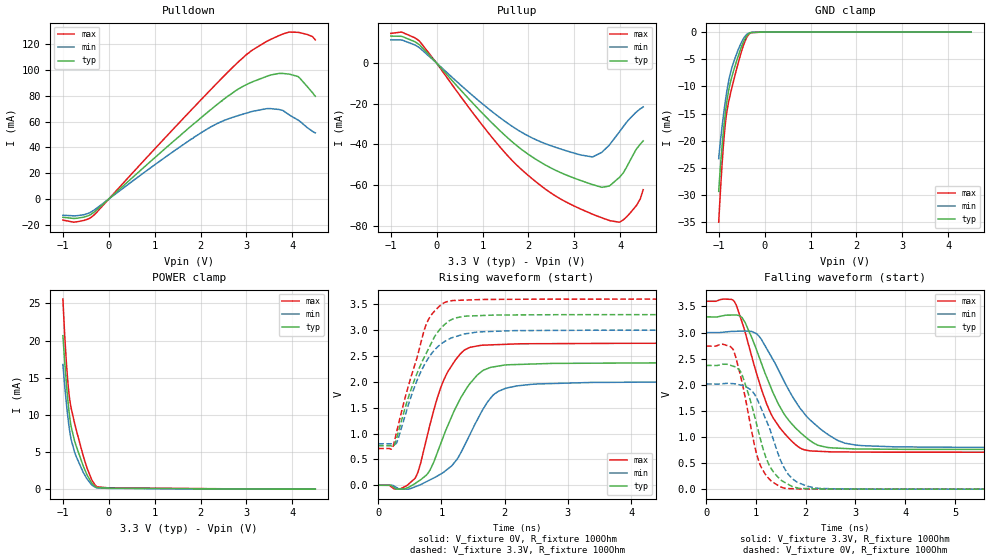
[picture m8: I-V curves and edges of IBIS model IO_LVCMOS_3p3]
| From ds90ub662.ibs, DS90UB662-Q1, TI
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|   IO_LVCMOS_3p3 Model
[Model]   IO_LVCMOS_3p3
Model_type   I/O
Polarity   Non-Inverting
Enable   Active-Low
Vinl = 0.99
Vinh = 2.31
Vmeas = 1.65
Vref = 0
Cref = 1pF
Rref = 100000
|   typ   min   max
C_comp   0.362pF   0.313pF   0.461pF
[Voltage Range]   3.3   3   3.6
[Temperature Range]   27   105   -40
[Pullup Reference]   3.3   3   3.6
[Pulldown Reference]   0   0   0
[Power Clamp Reference]   3.3   3   3.6
[GND Clamp Reference]   0   0   0
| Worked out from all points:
|   slope of the pulldown table from 0 to 0.495 V, typ, clamps not added: 31.1 ohm
|   slope of the pullup table from 0 to 0.495 V, typ, clamps not added: 39.6 ohm
|   GND clamp passes 1 mA (typ) near -0.41 V on its own axis
|   POWER clamp passes 1 mA (typ) near -0.39 V on its own axis
|   falling waveform, V_fixture 3.3V, R_fixture 100Ohm: 20-80 % time 741ps typ, 895ps min, 623ps max; typ from 3.3 V to 0.76 V
|   rising waveform, V_fixture 0V, R_fixture 100Ohm: 20-80 % time 524ps typ, 549ps min, 407ps max; typ from 0 V to 2.37 V
|   rising waveform, V_fixture 3.3V, R_fixture 100Ohm: 20-80 % time 485ps typ, 453ps min, 391ps max; typ from 0.764 V to 3.3 V
|   falling waveform, V_fixture 0V, R_fixture 100Ohm: 20-80 % time 435ps typ, 495ps min, 369ps max; typ from 2.37 V to 0 V
[Pulldown]
|   Voltage   I(typ)   I(min)   I(max)
-1V       -14.12mA   -12.57mA   -16.32mA
-686.5mV  -14.88mA   -12.9mA    -17.62mA
-318mV    -10.15mA   -8.516mA   -12.27mA
1.855V    58.36mA    47.77mA    71.05mA
2.432V    75.17mA    59.59mA    92.43mA
3.015V    88.88mA    66.66mA    112.2mA
3.532V    96.06mA    69.97mA    123.7mA
3.785V    97.25mA    68.67mA    127.7mA
3.933V    96.69mA    65.11mA    129.3mA
4.159V    93.73mA    60.33mA    128.8mA
4.439V    82.29mA    52.38mA    125.8mA
4.5V      79.54mA    51.15mA    123.2mA
[GND Clamp]
|   Voltage   I(typ)   I(min)   I(max)
-1V       -29.31mA   -23.3mA    -34.99mA
-950.5mV  -23.37mA   -19.11mA   -27.5mA
-901mV    -18.52mA   -15.58mA   -21.18mA
-862.5mV  -15.41mA   -13.12mA   -17.39mA
-818.5mV  -12.52mA   -10.64mA   -14.42mA
-780mV    -10.59mA   -8.845mA   -12.67mA
-736mV    -8.943mA   -7.241mA   -11.02mA
-576.5mV  -4.426mA   -3.263mA   -5.722mA
-488.5mV  -2.35mA    -1.606mA   -3.145mA
-406mV    -889.5uA   -555.3uA   -1.243mA
-312.5mV  -140.3uA   -92.62uA   -191.7uA
4.5V      0A         0A         0A
[Pullup]
|   Voltage   I(typ)   I(min)   I(max)
-1V       13.14mA    11.28mA    14.47mA
-774.5mV  13.05mA    11.25mA    15.11mA
-373mV    8.825mA    7.385mA    10.62mA
914mV     -22.78mA   -18.52mA   -28.24mA
1.53V     -36.43mA   -29.35mA   -45.12mA
2.223V    -48.15mA   -38.29mA   -59.41mA
2.839V    -55.13mA   -43.21mA   -68.45mA
3.394V    -59.68mA   -46.14mA   -74.2mA
3.752V    -60.44mA   -40.54mA   -77.2mA
4.066V    -53.93mA   -31.24mA   -77.01mA
4.362V    -41.98mA   -23.87mA   -69.58mA
4.5V      -38.24mA   -21.59mA   -62.21mA
[POWER Clamp]
|   Voltage   I(typ)   I(min)   I(max)
-1V       20.66mA    16.78mA    25.6mA
-961.5mV  17.23mA    14mA       20.8mA
-917.5mV  13.76mA    11.15mA    16.45mA
-884.5mV  11.52mA    9.313mA    13.9mA
-868mV    10.55mA    8.514mA    12.9mA
-829.5mV  8.747mA    6.995mA    11.22mA
-714mV    5.881mA    4.456mA    8.101mA
-565.5mV  3.265mA    2.379mA    4.665mA
-483mV    2.052mA    1.464mA    3.016mA
-356.5mV  701uA      495uA      1.09mA
-257.5mV  229.6uA    181.1uA    331.5uA
4.5V      0A         0A         0A
[Ramp]
R_load = 100
|   typ   min   max
dV/dt_r   1.42426/5.23477e-10   1.20925/5.45276e-10   1.64814/4.05887e-10
dV/dt_f   1.52372/7.39624e-10   1.32025/8.8776e-10   1.73603/6.1806e-10
[Falling Waveform]
V_fixture = 3.3V
V_fixture_min = 3V
V_fixture_max = 3.6V
R_fixture = 100Ohm
C_fixture = 0F
|   Time   V(typ)   V(min)   V(max)
0s        3.3V       3V         3.6V
538.9ps   3.335V     3.022V     3.623V
720.9ps   3.289V     3.028V     3.201V
1.02ns    2.649V     2.972V     2.196V
1.297ns   1.958V     2.56V      1.455V
1.606ns   1.385V     1.994V     1.035V
2.04ns    964.8mV    1.373V     740.9mV
2.789ns   779.1mV    880.4mV    712.4mV
3.795ns   764.4mV    810.4mV    707.8mV
20ns      760.4mV    799.5mV    706.5mV
[Rising Waveform]
V_fixture = 0V
V_fixture_min = 0V
V_fixture_max = 0V
R_fixture = 100Ohm
C_fixture = 0F
|   Time   V(typ)   V(min)   V(max)
0s        4.768uV    10.52uV    2.538uV
347.6ps   -75.13mV   -75.62mV   -69.45mV
577.1ps   27.84mV    -33.43mV   126.4mV
818.3ps   291.3mV    103.4mV    1.171V
1.07ns    1.067V     285.8mV    2.123V
1.352ns   1.783V     736.9mV    2.603V
1.614ns   2.178V     1.374V     2.704V
1.901ns   2.305V     1.816V     2.72V
2.526ns   2.347V     1.959V     2.737V
20ns      2.374V     2.015V     2.747V
[Rising Waveform]
V_fixture = 3.3V
V_fixture_min = 3V
V_fixture_max = 3.6V
R_fixture = 100Ohm
C_fixture = 0F
|   Time   V(typ)   V(min)   V(max)
0s        763.6mV    802.3mV    710.8mV
225.9ps   752.6mV    801.4mV    717.5mV
294.1ps   920.3mV    825.1mV    1.042V
499ps     1.781V     1.639V     2.01V
756.6ps   2.543V     2.386V     3.103V
912.3ps   2.915V     2.644V     3.395V
1.164ns   3.205V     2.852V     3.569V
1.564ns   3.278V     2.962V     3.588V
2.158ns   3.293V     2.99V      3.596V
20ns      3.3V       3V         3.6V
[Falling Waveform]
|Gnd
V_fixture = 0V
V_fixture_min = 0V
V_fixture_max = 0V
R_fixture = 100Ohm
C_fixture = 0F
|   Time   V(typ)   V(min)   V(max)
0s        2.37V      2.015V     2.741V
538.9ps   2.357V     2.021V     2.683V
737ps     2.153V     1.986V     1.983V
967.9ps   1.421V     1.825V     858.8mV
1.07ns    1.037V     1.628V     503.1mV
1.277ns   441.9mV    1.16V      186.8mV
1.578ns   130.5mV    393.9mV    16.82mV
1.84ns    22.8mV     128.2mV    4.699mV
2.598ns   2.593mV    5.842mV    1.211mV
20ns      5.193uV    11.53uV    2.627uV
